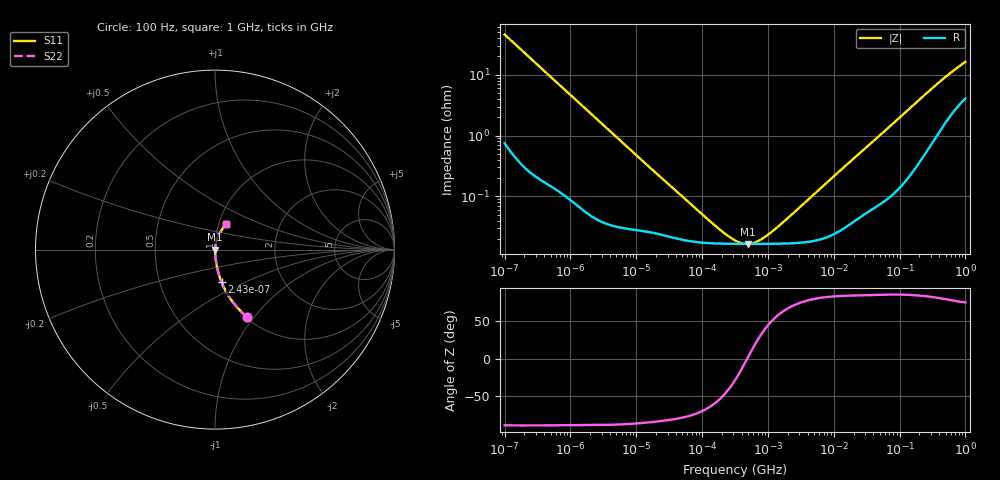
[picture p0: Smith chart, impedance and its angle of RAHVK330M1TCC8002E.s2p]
! RAHVK330M1TCC8002E  S-PARAMETER MODEL  (AEC-Q200 qualified)
! Model Generated by ELNA Corporation (http://www.ty-top.com)
! Version 1.0
! ELNA Control No. 201210
! Copyright (c) 2020 ELNA CO.,LTD. All Rights Reserved.
! Products Name : CONDUCTIVE POLYMER HYBRID ALUMINUM ELECTROLYTIC CAPACITORS
! Characteristics :
!  Capacitance  :  33uF  ,  Rated voltage  :  25V
!  Operating Temp. Range  :  -55 to +125 degC  ,  Endurance  :  4000hr at 125 degC
!  Dimension D  :  5mm  ,  Dimension L  :  5.8mm
! Frequency Range : 100Hz - 1GHz
! External Node Assignments :
!  1  o---| |---o  2
# MHz S RI R 50
!Freq[MHz].  S11 Real  S11 Imag  S21 Real  S21 Imag  S12 Real  S12 Imag  S22 Real  S22 Imag
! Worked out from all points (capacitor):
!   401 points, 100 Hz to 1 GHz, reference 50 ohm
!   read as one part in series: C = 34.7 uF near 108 Hz
!   lowest |Z| = 16.6 mohm at 492.6 kHz (marker M1)
!   series resonance near 483.2 kHz, so ESL is about 3.1 nH
!   S11 on the Smith chart (normalised r, x): 100 Hz: 1.01, -0.92; 243 Hz: 1.00, -0.38; 1 GHz: 1.08, +0.32
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0.0001  0.1781 -0.3745  0.8219 0.3745  0.8219 0.3745  0.1781 -0.3745
0.000113  0.1458 -0.3454  0.8542 0.3454  0.8542 0.3454  0.1458 -0.3454
0.000162  0.0772 -0.2604  0.9228 0.2604  0.9228 0.2604  0.0772 -0.2604
0.000243  0.0369 -0.1821  0.9631 0.1821  0.9631 0.1821  0.0369 -0.1821
0.000543  0.00855 -0.0843  0.9915 0.0843  0.9915 0.0843  0.00855 -0.0843
0.001488  0.0016 -0.0313  0.9984 0.0313  0.9984 0.0313  0.0016 -0.0313
0.004241  0.000454 -0.0111  0.9995 0.0111  0.9995 0.0111  0.000454 -0.0111
0.022131  0.000245 -0.00217  0.9998 0.00217  0.9998 0.00217  0.000245 -0.00217
0.159404  0.000169 -0.00028  0.9998 0.00028  0.9998 0.00028  0.000169 -0.00028
0.238506  0.000167 -0.000159  0.9998 0.000159  0.9998 0.000159  0.000167 -0.000159
0.316228  0.000166 -9.08e-05  0.9998 9.08e-05  0.9998 9.08e-05  0.000166 -9.08e-05
0.402717  0.000166 -3.81e-05  0.9998 3.81e-05  0.9998 3.81e-05  0.000166 -3.81e-05
0.492606  0.000165 4.07e-06  0.9998 -4.07e-06  0.9998 -4.07e-06  0.000165 4.07e-06
0.679986  0.000165 7.25e-05  0.9998 -7.25e-05  0.9998 -7.25e-05  0.000165 7.25e-05
1.017419  0.000166 0.00017  0.9998 -0.00017  0.9998 -0.00017  0.000166 0.00017
1.717908  0.000167 0.000341  0.9998 -0.000341  0.9998 -0.000341  0.000167 0.000341
4.704354  0.000184 0.001  0.9998 -0.001  0.9998 -0.001  0.000184 0.001
69.9842  0.00115 0.0138  0.9988 -0.0138  0.9988 -0.0138  0.00115 0.0138
176.8072  0.00413 0.0342  0.9959 -0.0342  0.9959 -0.0342  0.00413 0.0342
395.8221  0.0163 0.0718  0.9837 -0.0718  0.9837 -0.0718  0.0163 0.0718
695.825  0.0388 0.1119  0.9612 -0.1119  0.9612 -0.1119  0.0388 0.1119
1000  0.0608 0.1426  0.9392 -0.1426  0.9392 -0.1426  0.0608 0.1426
